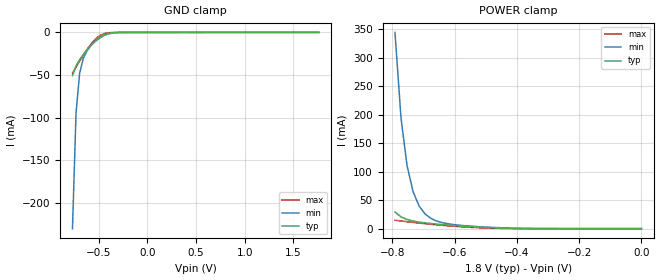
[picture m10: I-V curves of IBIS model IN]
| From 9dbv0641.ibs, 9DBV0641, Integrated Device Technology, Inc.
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|   Model IN
[Model]   IN
Model_type   Input
Polarity   Non-Inverting
Vinl = 0.63V
Vinh = 1.17V
|   typ   min   max
C_comp   2pF   1.5pF   2.5pF
|   typ   min   max
[Voltage range]   1.8V   1.7V   1.9V
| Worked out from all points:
|   GND clamp passes 1 mA (typ) near -0.39 V on its own axis
|   POWER clamp passes 1 mA (typ) near -0.45 V on its own axis
[GND_clamp]
|Voltage   I (typ)   I (min)   I (max)
|Note, modeling breaks down at 250mA and above.  This is well beyond the functional   |
|operating range of the device.  Should this scenario occur, catastrophic failure and   |
|possible damage to the device and/or board is of higher concern than the I-V curve   |
|behavior.  The IBIS checker will flag currents in excess of 10A with warnings.  Lines   |
|with currents in excess of 0.35 A have been commented out.  The points still remain|
|available to the user if the user desires to use them.   |
|-1.80000e+00   -4.43726e+01   -4.17458e+01   -4.86820e+01
|-1.76327e+00   -4.25922e+01   -4.02056e+01   -4.65395e+01
|-1.72653e+00   -4.08117e+01   -3.86654e+01   -4.43969e+01
|-1.68980e+00   -3.90312e+01   -3.71251e+01   -4.22544e+01
|-1.65306e+00   -3.72507e+01   -3.55849e+01   -4.01118e+01
|-1.61633e+00   -3.54702e+01   -3.40446e+01   -3.79693e+01
|-1.57959e+00   -3.36896e+01   -3.25043e+01   -3.58267e+01
|-1.54286e+00   -3.19091e+01   -3.09640e+01   -3.36840e+01
|-1.50612e+00   -3.01285e+01   -2.94236e+01   -3.15414e+01
|-1.46939e+00   -2.83479e+01   -2.78833e+01   -2.93987e+01
|-1.43265e+00   -2.65672e+01   -2.63429e+01   -2.72561e+01
|-1.39592e+00   -2.47866e+01   -2.48025e+01   -2.51134e+01
|-1.35918e+00   -2.30059e+01   -2.32621e+01   -2.29707e+01
|-1.32245e+00   -2.12253e+01   -2.17217e+01   -2.08279e+01
|-1.28571e+00   -1.94446e+01   -2.01813e+01   -1.86852e+01
|-1.24898e+00   -1.76639e+01   -1.86409e+01   -1.65424e+01
|-1.21224e+00   -1.58832e+01   -1.71005e+01   -1.43996e+01
|-1.17551e+00   -1.41025e+01   -1.55600e+01   -1.22568e+01
|-1.13878e+00   -1.23218e+01   -1.40196e+01   -1.01141e+01
|-1.10204e+00   -1.05411e+01   -1.24792e+01   -7.97124e+00
|-1.06531e+00   -8.76046e+00   -1.09388e+01   -5.82843e+00
|-1.02857e+00   -6.97978e+00   -9.39848e+00   -3.68562e+00
|-9.91837e-01   -5.19912e+00   -7.85813e+00   -1.54785e+00
|-9.55102e-01   -3.41847e+00   -6.31781e+00   -3.90595e-01
|-9.18367e-01   -1.63807e+00   -4.77753e+00   -1.29996e-01
|-8.81633e-01   -5.21907e-01   -3.23728e+00   -7.87800e-02
|-8.44898e-01   -1.73459e-01   -1.69709e+00   -6.40873e-02
|-8.08163e-01   -7.85613e-02   -6.33127e-01   -5.54276e-02
-771.4mV  -50.63mA   -230.2mA   -47.85mA
-734.7mV  -39.27mA   -94.07mA   -40.58mA
-698mV    -32.06mA   -48.05mA   -33.55mA
-661.2mV  -26.07mA   -30.55mA   -26.83mA
-624.5mV  -20.62mA   -22.01mA   -20.51mA
-587.8mV  -15.64mA   -16.46mA   -14.75mA
-514.3mV  -7.457mA   -8.514mA   -5.771mA
-477.6mV  -4.509mA   -5.592mA   -2.97mA
-404.1mV  -1.167mA   -1.846mA   -517.4uA
-293.9mV  -74.63uA   -181.5uA   -23.43uA
1.763V    14.13uA    10.16uA    21.47uA
[Power_clamp]
|Voltage   I (typ)   I (min)   I (max)
|Note, modeling breaks down at 250mA and above.  This is well beyond the functional   |
|operating range of the device.  Should this scenario occur, catastrophic failure and   |
|possible damage to the device and/or board is of higher concern than the I-V curve   |
|behavior.  The IBIS checker will flag currents in excess of 10A with warnings.  Lines   |
|with currents in excess of 0.35 A have been commented out.  The points still remain|
|available to the user if the user desires to use them.   |
|-1.80000e+00   5.60662e+01   5.31750e+01   6.07752e+01
|-1.78061e+00   5.48637e+01   5.21252e+01   5.93477e+01
|-1.76122e+00   5.36611e+01   5.10754e+01   5.79201e+01
|-1.74184e+00   5.24586e+01   5.00255e+01   5.64925e+01
|-1.72245e+00   5.12561e+01   4.89757e+01   5.50649e+01
|-1.70306e+00   5.00535e+01   4.79259e+01   5.36374e+01
|-1.68367e+00   4.88510e+01   4.68761e+01   5.22098e+01
|-1.66429e+00   4.76485e+01   4.58263e+01   5.07822e+01
|-1.64490e+00   4.64460e+01   4.47765e+01   4.93547e+01
|-1.62551e+00   4.52434e+01   4.37267e+01   4.79271e+01
|-1.60612e+00   4.40409e+01   4.26769e+01   4.64996e+01
|-1.58673e+00   4.28384e+01   4.16272e+01   4.50720e+01
|-1.56735e+00   4.16359e+01   4.05774e+01   4.36444e+01
|-1.54796e+00   4.04334e+01   3.95276e+01   4.22169e+01
|-1.52857e+00   3.92308e+01   3.84778e+01   4.07893e+01
|-1.50918e+00   3.80283e+01   3.74280e+01   3.93618e+01
|-1.48980e+00   3.68258e+01   3.63783e+01   3.79342e+01
|-1.47041e+00   3.56233e+01   3.53285e+01   3.65067e+01
|-1.45102e+00   3.44208e+01   3.42787e+01   3.50791e+01
|-1.43163e+00   3.32183e+01   3.32290e+01   3.36516e+01
|-1.41224e+00   3.20159e+01   3.21792e+01   3.22241e+01
|-1.39286e+00   3.08134e+01   3.11294e+01   3.07965e+01
|-1.37347e+00   2.96109e+01   3.00797e+01   2.93690e+01
|-1.35408e+00   2.84084e+01   2.90300e+01   2.79415e+01
|-1.33469e+00   2.72059e+01   2.79802e+01   2.65140e+01
|-1.31531e+00   2.60035e+01   2.69305e+01   2.50865e+01
|-1.29592e+00   2.48010e+01   2.58808e+01   2.36589e+01
|-1.27653e+00   2.35986e+01   2.48310e+01   2.22314e+01
|-1.25714e+00   2.23961e+01   2.37813e+01   2.08039e+01
|-1.23776e+00   2.11937e+01   2.27316e+01   1.93764e+01
|-1.21837e+00   1.99912e+01   2.16819e+01   1.79490e+01
|-1.19898e+00   1.87888e+01   2.06322e+01   1.65215e+01
|-1.17959e+00   1.75864e+01   1.95825e+01   1.50940e+01
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-791.8mV  29.26mA    344.8mA    14.84mA
-772.4mV  20.73mA    194.3mA    13.49mA
-753.1mV  16.1mA     110.7mA    12.21mA
-733.7mV  13.35mA    64.84mA    10.99mA
-714.3mV  11.49mA    39.63mA    9.831mA
-694.9mV  10.08mA    25.65mA    8.721mA
-675.5mV  8.904mA    17.72mA    7.666mA
-636.7mV  6.907mA    10.16mA    5.729mA
-539.8mV  3.07mA     4.093mA    2.051mA
-365.3mV  167.9uA    383.5uA    57.09uA
0V        14.13nA    10.08nA    21.48nA
